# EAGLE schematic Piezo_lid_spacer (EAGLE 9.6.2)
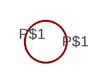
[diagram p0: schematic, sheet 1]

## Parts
U$5  SPRING_PAD  [SPRING_PAD]
Unconnected: U$5.P$1

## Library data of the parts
U$5 = RGB_library:SPRING_PAD

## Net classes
1 connect: width 0.457 mm, clearance 0.152 mm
